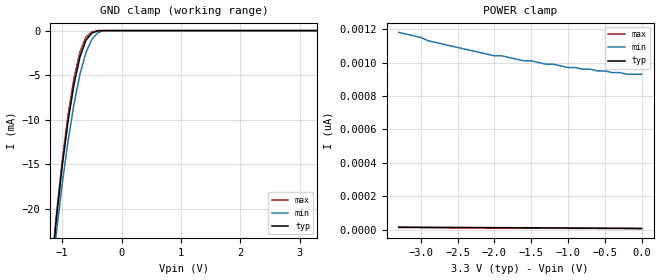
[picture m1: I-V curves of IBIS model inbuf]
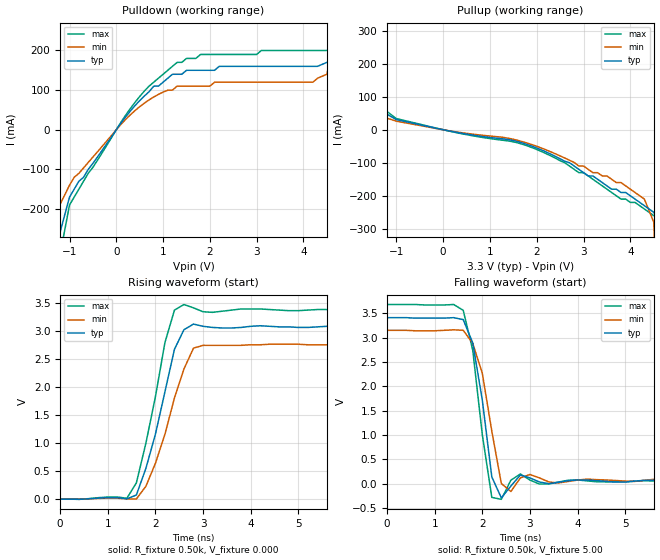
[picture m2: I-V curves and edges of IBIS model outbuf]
| IBIS file 43807.ibs created by s2ibis2 version 1.1
| North Carolina State University Electronics Research Laboratory  1995
[IBIS ver]   2.1
[File name]   43807.ibs
[File Rev]   0.1
[Date]   Wednesday, March 12, 1997
[Source]   IDT
[Notes]   1. Temp typ=25C, min=100C, max=0C 2. Ramp rates based on 500
   ohm load
[Copyright]   Copyright 1997, Integrated Device Technology, Inc.
[Disclaimer] Integrated Device Technology, Inc. ("IDT") hereby grants the
   user of this IBIS model a non-exclusive, nontransferable
   license to use this IBIS model under the following terms.
   The user is granted this license only to use the IBIS model
   and is not granted rights to sell, copy (except as needed to
   run the IBIS model), rent, lease or sub-license the IBIS model
   in whole or in part, or in modified form to anyone.
   The User may modify the IBIS model to suit its specific
   applications, but rights to derivative works and such
   modifications shall belong to IDT.
   This IBIS model is provided on an "AS IS" basis and IDT
   makes absolutely no warranty with respect to the information
   contained herein. IDT DISCLAIMS AND CUSTOMER WAIVES ALL
   WARRANTIES, EXPRESS AND IMPLIED, INCLUDING WARRANTIES OF
   MERCHANTABILITY AND FITNESS FOR A PARTICULAR PURPOSE. THE
   ENTIRE RISK AS TO QUALITY AND PERFORMANCE IS WITH THE
   USER ACCORDINGLY, IN NO EVENT SHALL IDT BE LIABLE
   FOR ANY DIRECT OR INDIRECT DAMAGES, WHETHER IN CONTRACT OR
   TORT, INCLUDING ANY LOST PROFITS OR OTHER INCIDENTAL,
   CONSEQUENTIAL, EXEMPLARY, OR PUNITIVE DAMAGES ARISING OUT OF
   THE USE OR APPLICATION OF THE IBIS model.  Further, IDT
   reserves the right to make changes without notice to any
   product herein to improve reliability, function, or design.
   IDT does not convey any license under patent rights or
   any other intellectual property rights, including those of
   third parties. IDT is not obligated to provide maintenance
   or support for the licensed IBIS model.
|   COMPONENT: IDT74FCT3807/A
[Component]   IDT74FCT3807/A
[Manufacturer]   Integrated Device Technology Inc.
[Package]
| SO20-2 SSOP
| variable   typ   min   max
R_pkg   10.00m   9.00m   11.00m
L_pkg   3.50nH   3.00nH   4.00nH
C_pkg   0.30pF   0.26pF   0.34pF
[Pin]  signal_name   model_name   R_pin  L_pin  C_pin
1   IN   inbuf
2   GND   GND
3   O1   outbuf
4   VCC   POWER
5   O2   outbuf
6   GND   GND
7   O3   outbuf
8   VCC   POWER
9   O4   outbuf
10   GND   GND
11   O5   outbuf
12   O6   outbuf
13   GND   GND
14   O7   outbuf
15   VCC   POWER
16   O8   outbuf
17   GND   GND
18   O9   outbuf
19   O10   outbuf
20   VCC   POWER
| Models and submodels in the file (2): inbuf (Input), outbuf (Output)
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|   Model inbuf
[Model]   inbuf
Model_type   Input
Vinl =   0.80V
Vinh =   2.00V
C_comp   5.00pF   5.00pF   5.00pF
[Temperature Range]   25.00   100.00   0.000
[Voltage Range]   3.30V   3.00V   3.60V
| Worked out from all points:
|   GND clamp passes 1 mA (typ) near -0.59 V on its own axis
[GND_clamp]
| voltage   I(typ)   I(min)   I(max)
-3.3V     -32.08A    -29.15A    -33.09A
-1.2V     -28.45mA   -29.36mA   -28.25mA
-1.1V     -21.32mA   -22.89mA   -20.85mA
-1V       -15.28mA   -17.27mA   -14.63mA
-900mV    -10.16mA   -12.37mA   -9.41mA
-800mV    -6.02mA    -8.22mA    -5.29mA
-700mV    -2.96mA    -4.9mA     -2.36mA
-600mV    -1.08mA    -2.48mA    -720uA
-500mV    -290uA     -990uA     -150uA
-400mV    -19.55uA   -240uA     -5.7uA
-300mV    -240nA     -9.44uA    -45.73nA
3.3V      8.95pA     940pA      6.75pA
[POWER_clamp]
| voltage   I(typ)   I(min)   I(max)
-3.3V     16.3pA     1.18nA     14pA
-3V       15.6pA     1.15nA     13.4pA
-2.9V     15.36pA    1.13nA     13.2pA
-2V       13.31pA    1.04nA     11.38pA
-1.9V     13.1pA     1.04nA     11.19pA
-1.6V     12.42pA    1.01nA     10.59pA
-1.5V     12.19pA    1.01nA     10.37pA
-1.3V     11.75pA    990pA      9.97pA
-1.2V     11.54pA    990pA      9.77pA
-1V       11.1pA     970pA      9.37pA
-200mV    9.38pA     930pA      7.76pA
0V        8.95pA     930pA      7.36pA
|   Model outbuf
[Model]   outbuf
Model_type   Output
Polarity   Non-Inverting
C_comp   5.00pF   5.00pF   5.00pF
[Temperature Range]   25.00   100.00   0.000
[Voltage Range]   3.30V   3.00V   3.60V
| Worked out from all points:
|   slope of the pulldown table from 0 to 0.495 V, typ, clamps not added: 6.79 ohm
|   slope of the pullup table from 0 to 0.495 V, typ, clamps not added: 37.7 ohm
|   rising waveform, R_fixture 0.50k, V_fixture 0.000: 20-80 % time 522ps typ, 596ps min, 471ps max; typ from 0 V to 3.08 V
|   falling waveform, R_fixture 0.50k, V_fixture 5.00: 20-80 % time 299ps typ, 359ps min, 288ps max; typ from 3.41 V to 0.063 V
[Pulldown]
| voltage   I(typ)   I(min)   I(max)
-3.3V     -40.26A    -36.59A    -41.52A
-1.5V     -390mA     -260mA     -500mA
-900mV    -150mA     -120mA     -170mA
100mV     16.97mA    13.72mA    19.08mA
800mV     110mA      82.66mA    120mA
1.3V      140mA      110mA      170mA
4.2V      160mA      120mA      200mA
4.5V      170mA      140mA      200mA
4.7V      170mA      260mA      200mA
4.9V      290mA      590mA      210mA
5.1V      650mA      1.03A      260mA
6.6V      4.49A      4.89A      3.85A
[Pullup]
| voltage   I(typ)   I(min)   I(max)
-3.3V     4.32A      3.96A      4.44A
-1.9V     710mA      480mA      800mA
-1.7V     300mA      160mA      360mA
-1.5V     71.08mA    48.65mA    87.28mA
-1V       30.66mA    25.86mA    33.78mA
2.2V      -67.32mA   -61.01mA   -72.36mA
3.8V      -190mA     -160mA     -210mA
4.3V      -230mA     -210mA     -240mA
4.5V      -250mA     -280mA     -260mA
4.7V      -300mA     -980mA     -280mA
4.9V      -950mA     -3.65A     -310mA
6.6V      -40.3A     -44.23A    -33.89A
[Ramp]
| variable   typ   min   max
dV/dt_r   1.85/0.51n   1.66/0.58n   2.03/0.46n
dV/dt_f   1.96/0.27n   1.77/0.29n   2.14/0.25n
R_load = 0.50k
[Rising Waveform]
R_fixture = 0.50k
V_fixture = 0.000
| time   V(typ)   V(min)   V(max)
0s        0V         0V         0V
1.4ns     5.47mV     5.4mV      15.47mV
1.6ns     73.89mV    2.67mV     290mV
1.8ns     550mV      230mV      1V
2.2ns     1.92V      1.16V      2.8V
2.4ns     2.68V      1.81V      3.38V
2.6ns     3.03V      2.33V      3.48V
2.8ns     3.13V      2.7V       3.42V
3ns       3.09V      2.75V      3.35V
10ns      3.08V      2.76V      3.38V
[Falling Waveform]
R_fixture = 0.50k
V_fixture = 5.00
| time   V(typ)   V(min)   V(max)
0s        3.41V      3.15V      3.68V
1.6ns     3.37V      3.15V      3.56V
1.8ns     2.89V      2.88V      2.74V
2ns       1.72V      2.27V      1.01V
2.2ns     140mV      1.08V      -280mV
2.4ns     -290mV     5.1mV      -320mV
2.6ns     -47.72mV   -160mV     73.06mV
3ns       120mV      190mV      75.4mV
3.6ns     29.93mV    16.44mV    34.6mV
10ns      62.99mV    77.02mV    53.78mV
